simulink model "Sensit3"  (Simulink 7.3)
settings: Solver=ode45  StartTime=0.0  StopTime=30  RelTol=1e-3
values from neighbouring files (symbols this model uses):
  Kp = om^2    (= 1.44)    [run.m]
  Kp3 = [0.3042  3.4539  0.5105  0.0711 -0.2670]    [run.m]
  Kr = 2*zt*om    (= 0.336)    [run.m]
undefined symbols (not defined in the file or in its folder): An, Bn, Cn, Dn

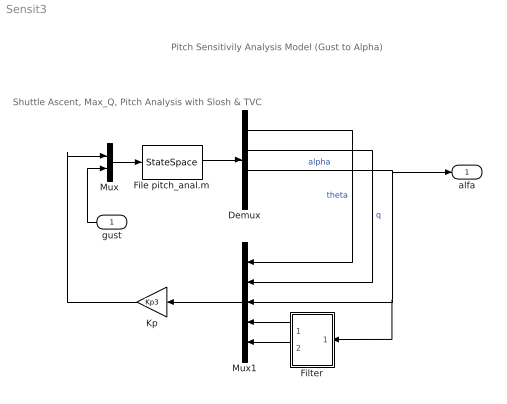
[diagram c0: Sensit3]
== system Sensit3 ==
  note: Pitch Sensitivily Analysis Model (Gust to Alpha)
  note: Shuttle Ascent, Max_Q, Pitch Analysis with Slosh & TVC
  gust : Inport  OutDataType=sfix(16)  OutScaling=2^0
  Demux : Demux
  File pitch_anal.m : StateSpace  A=An  B=Bn  C=Cn  D=Dn
  Filter : Subsystem
  Kp : Gain  Gain=Kp3  Multiplication=Matrix(K*u)  ParameterDataType=sfix(16)  ParameterScaling=2^0  OutDataType=sfix(16)  OutScaling=2^0
  Mux : Mux  Inputs=2
  Mux1 : Mux  Inputs=5
  alfa : Outport  OutDataType=sfix(16)  OutScaling=2^0
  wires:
  Mux/1 -> File pitch_anal.m/1
  Demux/2 -> Mux1/2  "q"
  Demux/1 -> Mux1/1  "theta"
  gust/1 -> Mux/2
  Kp/1 -> Mux/1
  File pitch_anal.m/1 -> Demux/1
  Mux1/1 -> Kp/1
  Filter/1(x1) -> Mux1/4
  Filter/2(x2) -> Mux1/5
  Demux/3 -> alfa/1, Filter/1(a), Mux1/3  "alpha"

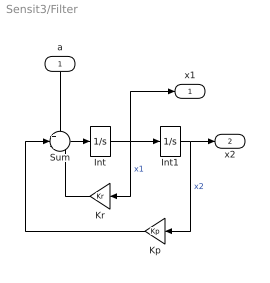
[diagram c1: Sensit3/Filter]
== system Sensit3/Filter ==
  a : Inport  OutDataType=sfix(16)  OutScaling=2^0
  Int : Integrator
  Int1 : Integrator
  Kp : Gain  Gain=Kp  ParameterDataType=sfix(16)  ParameterScaling=2^0  OutDataType=sfix(16)  OutScaling=2^0
  Kr : Gain  Gain=Kr  ParameterDataType=sfix(16)  ParameterScaling=2^0  OutDataType=sfix(16)  OutScaling=2^0
  Sum : Sum  Inputs=+--  OutDataType=sfix(16)  OutScaling=2^0
  x1 : Outport  OutDataType=sfix(16)  OutScaling=2^0
  x2 : Outport  Port=2  OutDataType=sfix(16)  OutScaling=2^0
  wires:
  Int/1 -> Int1/1, Kr/1, x1/1  "x1"
  Sum/1 -> Int/1
  Int1/1 -> Kp/1, x2/1  "x2"
  Kr/1 -> Sum/3
  Kp/1 -> Sum/2
  a/1 -> Sum/1
